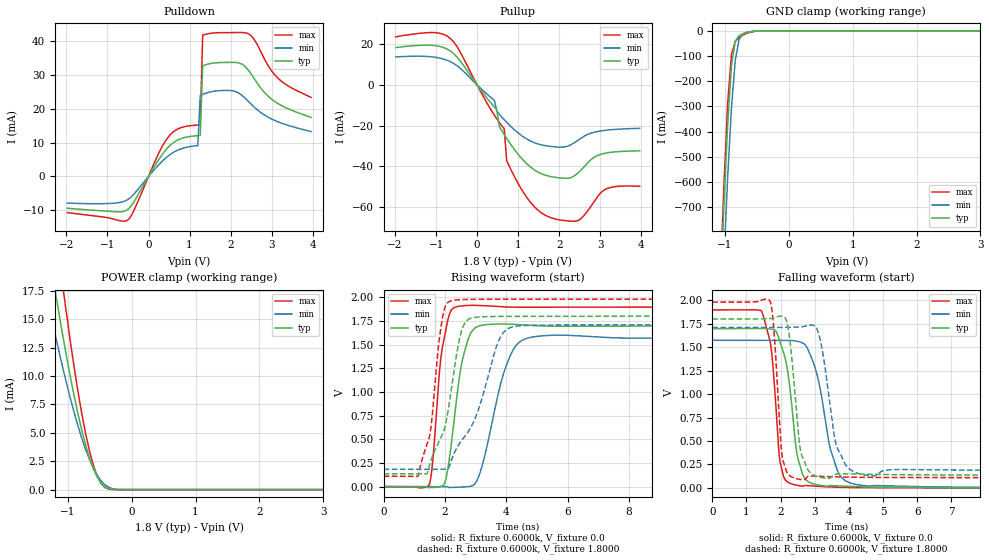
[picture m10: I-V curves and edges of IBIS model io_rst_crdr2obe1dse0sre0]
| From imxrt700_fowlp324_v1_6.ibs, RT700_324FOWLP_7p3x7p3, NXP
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[Model] io_rst_crdr2obe1dse0sre0
|   Model io_rst_crdr2obe1dse0sre0
| This model was characterised for following simulation conditions:
| External (pad) voltage:
|   - Typ: 1.8V,   - Min: 1.71V,   - Max: 1.98V
| Library cells for typ/min/max conditions are connected as defined below:
|  PAD_RST - External Pad
|  ipp_do - Core Input
|  ipp_obe - Output Buffer Enable
|  ASRCN3V3[3] - NC
|  ASRCN3V3[4] - NC
|  ASRCP3V3[4] - NC
|  REFAPBIAS3V3 - gnde
|  REFBAMPL3V3 - vdd1v8
|  REFCAMPH3V3 - vdd1v8
|  REFDNBIAS3V3 - vdd1v8
|  REFH3V3 - REFH3V3
|  REFL3V3 - REFL3V3
|  gnde - gnde
|  ipp_dse - gnde
|  ipp_ina235_3v - NC
|  ipp_ina40_3v - NC
|  ipp_ina_mux - NC
|  ipp_ind - NC
|  ipp_ind_1p8v - NC
|  ipp_ind_3v - NC
|  ipp_sre - gnde
|  vdd - vdd
|  vdd1v8 - vdd1v8
|  vdda - vdde3v3
|  vdde3v3 - vdde3v3
| All other pins connected to ground
Model_type I/O
Polarity   Non-Inverting
Enable   Active-High
Vinl =   0.5400V
Vinh =   1.2600V
Vmeas =  0.9000V
Cref =   15.0000pF
Rref =   0.6000k
Vref =   0.0V
C_comp   3.9797pF   3.7947pF   4.1049pF
|C_comp_pullup   0.4869pF   0.5824pF   0.4755pF
|C_comp_pulldown   2.0823pF   2.1674pF   1.8519pF
[Model Spec]
| variable   typ   min   max
Vinh   1.2600V   NA   NA
Vinl   0.5400V   NA   NA
Vref   0.0V   0.0V   0.0V
Cref   15.0000pF   15.0000pF   15.0000pF
Rref   0.6000k   0.6000k   0.6000k
[Receiver Thresholds]
Vcross_high  =   0.0V
Vcross_low  =   0.0V
Vdiff_ac  =   0.0V
Vdiff_dc  =   0.0V
Tdiffslew_ac  =   0.0S
[Temperature Range]   25.0000   0.1250k   -40.0000
[Voltage Range]   1.8000V   1.7100V   1.9800V
[Pullup Reference]   1.8000V   1.7100V   1.9800V
[Pulldown Reference]   0.0V   0.0V   0.0V
[POWER Clamp Reference]   1.8000V   1.7100V   1.9800V
[GND Clamp Reference]   0.0V   0.0V   0.0V
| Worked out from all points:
|   slope of the pulldown table from 0 to 0.27 V, typ, clamps not added: 50.4 ohm
|   slope of the pullup table from 0 to 0.27 V, typ, clamps not added: 37.4 ohm
|   GND clamp passes 1 mA (typ) near -0.50 V on its own axis
|   POWER clamp passes 1 mA (typ) near -0.53 V on its own axis
|   rising waveform, R_fixture 0.6000k, V_fixture 0.0: 20-80 % time 421ps typ, 689ps min, 313ps max; typ from 0 V to 1.7 V
|   rising waveform, R_fixture 0.6000k, V_fixture 1.8000: 20-80 % time 623ps typ, 1.06ns min, 382ps max; typ from 0.135 V to 1.8 V
|   falling waveform, R_fixture 0.6000k, V_fixture 0.0: 20-80 % time 342ps typ, 520ps min, 239ps max; typ from 1.7 V to 0 V
|   falling waveform, R_fixture 0.6000k, V_fixture 1.8000: 20-80 % time 249ps typ, 359ps min, 184ps max; typ from 1.8 V to 0.135 V
[Pulldown]
|Voltage   I(typ)   I(min)   I(max)
-1.98V    -9.436mA   -7.894mA   -10.73mA
-480mV    -9.54mA    -6.639mA   -12.65mA
480mV     8.647mA    6.046mA    11.65mA
780mV     11.13mA    8.114mA    14.39mA
1.2V      12.06mA    9.104mA    15.21mA
1.26V     12.11mA    23.94mA    15.24mA
1.32V     32.75mA    24.29mA    41.84mA
2.04V     33.78mA    25.37mA    42.6mA
2.46V     31.05mA    21.88mA    42.06mA
2.82V     24.92mA    18.21mA    34.86mA
3.12V     21.84mA    16.34mA    29.51mA
3.96V     17.47mA    13.28mA    23.42mA
[Pullup]
|Voltage   I(typ)   I(min)   I(max)
-1.98V    18.38mA    13.75mA    23.61mA
-600mV    15.86mA    10.88mA    21.76mA
420mV     -10.83mA   -7.487mA   -14.84mA
480mV     -12.18mA   -12.88mA   -16.66mA
540mV     -20.35mA   -14.31mA   -18.38mA
660mV     -24.32mA   -17.04mA   -21.51mA
720mV     -26.22mA   -18.33mA   -37.1mA
900mV     -31.46mA   -21.85mA   -44.64mA
1.62V     -44.01mA   -29.64mA   -63.5mA
2.4V      -44.17mA   -27.97mA   -66.91mA
3.12V     -33.49mA   -22.27mA   -51.3mA
3.96V     -32.36mA   -21.3mA    -49.74mA
[GND_clamp]
|Voltage   I(typ)   I(min)   I(max)
-1.98V    -7.543A    -7.6A      -7.897A
-1.08V    -1.077A    -1.286A    -1.025A
-1.02V    -705.3mA   -921.3mA   -628.8mA
-960mV    -377.1mA   -587.4mA   -291.7mA
-900mV    -139.2mA   -307mA     -94.38mA
-840mV    -40.12mA   -117mA     -42.82mA
-780mV    -18.81mA   -33.95mA   -26.13mA
-720mV    -11.86mA   -11.44mA   -16.78mA
-660mV    -7.061mA   -5.737mA   -9.992mA
-540mV    -1.684mA   -1.901mA   -2.15mA
-420mV    -207.1uA   -403.7uA   -160.6uA
3.96V     0A         0A         0A
[POWER_clamp]
|Voltage   I(typ)   I(min)   I(max)
-1.98V    46.79mA    35.94mA    61.38mA
-1.32V    21.77mA    16.85mA    28.91mA
-1.2V     17.57mA    13.71mA    23.33mA
-1.14V    15.55mA    12.2mA     20.62mA
-1.08V    13.59mA    10.75mA    17.99mA
-1.02V    11.7mA     9.353mA    15.46mA
-900mV    8.209mA    6.76mA     10.73mA
-720mV    3.898mA    3.51mA     4.887mA
-540mV    1.103mA    1.267mA    1.195mA
-420mV    244.5uA    429.2uA    190.6uA
-180mV    280.9nA    5.273uA    26.8nA
3.96V     0A         0A         0A
[Ramp]
| variable   typ   min   max
dV/dt_r  1.0186/0.4212n   0.9439/0.6892n   1.1383/0.3125n
dV/dt_f  0.9990/0.2492n   0.9166/0.3588n   1.1224/0.1844n
R_load = 0.6000k
[Rising Waveform]
R_fixture= 0.6000k
V_fixture= 0.0
V_fixture_min= 0.0
V_fixture_max= 0.0
|time   V(typ)   V(min)   V(max)
0s        115.1nV    3.181uV    43.69nV
1.495ns   -9.973mV   -1.009mV   27.59mV
1.913ns   7.917mV    -887.7uV   1.467V
2.1ns     199.4mV    -4.399mV   1.77V
2.532ns   1.277V     -5.483mV   1.909V
2.799ns   1.593V     2.23mV     1.914V
3.112ns   1.696V     117.1mV    1.913V
4.168ns   1.715V     1.409V     1.895V
5.143ns   1.697V     1.592V     1.895V
60ns      1.698V     1.573V     1.897V
[Rising Waveform]
R_fixture= 0.6000k
V_fixture= 1.8000
V_fixture_min= 1.7100
V_fixture_max= 1.9800
|time   V(typ)   V(min)   V(max)
0s        135mV      182.4mV    109.3mV
1.122ns   134.2mV    182.3mV    111.8mV
1.522ns   255.2mV    181.5mV    573.7mV
1.78ns    458.4mV    181.8mV    1.464V
1.942ns   567.4mV    182.3mV    1.822V
2.364ns   1.367V     394.9mV    1.972V
2.767ns   1.766V     584.3mV    1.977V
3.808ns   1.798V     1.579V     1.979V
4.487ns   1.798V     1.7V       1.979V
60ns      1.8V       1.71V      1.98V
[Falling Waveform]
R_fixture= 0.6000k
V_fixture= 0.0
V_fixture_min= 0.0
V_fixture_max= 0.0
|time   V(typ)   V(min)   V(max)
0s        1.698V     1.573V     1.897V
1.443ns   1.699V     1.573V     1.882V
1.709ns   1.693V     1.573V     1.528V
1.87ns    1.667V     1.573V     838.6mV
2.083ns   1.446V     1.574V     127.4mV
2.615ns   175.8mV    1.549V     18.74mV
3.047ns   33.84mV    1.237V     16.84mV
3.689ns   21.28mV    165.6mV    6.716mV
4.577ns   9.605mV    19.47mV    2.259mV
60ns      6.624uV    14.17uV    1.076uV
[Falling Waveform]
R_fixture= 0.6000k
V_fixture= 1.8000
V_fixture_min= 1.7100
V_fixture_max= 1.9800
|time   V(typ)   V(min)   V(max)
0s        1.8V       1.71V      1.98V
1.693ns   1.804V     1.71V      1.99V
1.797ns   1.809V     1.709V     1.724V
2.058ns   1.829V     1.71V      307.9mV
2.241ns   1.661V     1.712V     139.1mV
2.646ns   325mV      1.718V     84.66mV
3.126ns   115.3mV    1.631V     123.4mV
3.674ns   148mV      414mV      116.1mV
4.646ns   144mV      127.8mV    111.4mV
60ns      135mV      182.4mV    109.3mV
